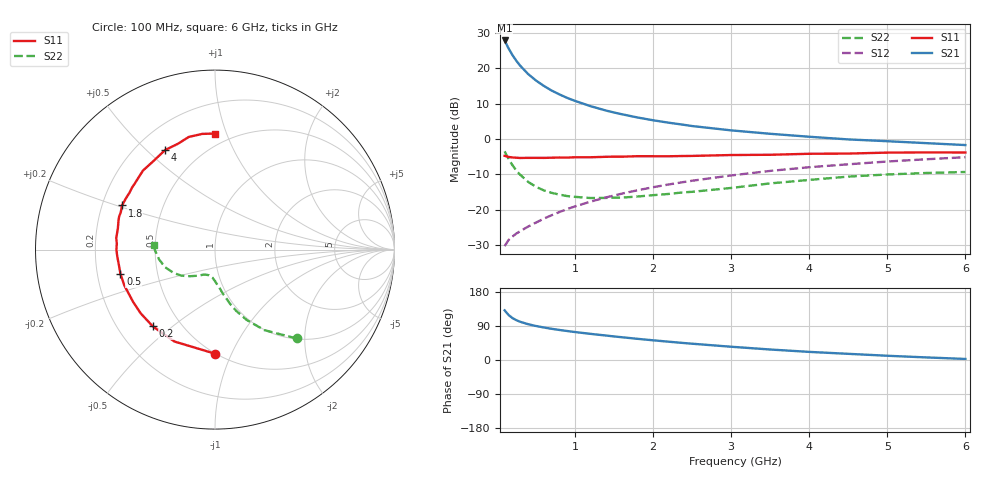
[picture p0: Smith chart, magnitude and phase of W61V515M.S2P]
! SIEMENS Small Signal Semiconductors
! BFR193W
! Si NPN RF Bipolar Junction Transistor in SOT323
! VCE = 1.5 V  IC = 15 mA
! Common Emitter S-Parameters:  September  1992
# GHz  S  MA  R  50
!  f  S11  S21  S12  S22
! GHz  MAG  ANG  MAG  ANG  MAG  ANG  MAG  ANG
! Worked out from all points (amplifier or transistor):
!   28 points, 100 MHz to 6 GHz, reference 50 ohm
!   highest |S21| = 27.9 dB at 100 MHz (marker M1)
!   |S21| within 3 dB of that: start of sweep to 170.7 MHz
!   unconditionally stable (mu >= 1): 809.9 MHz to 2.601 GHz
!   at 300 MHz: K = 0.69, MSG = 23.4 dB, |S12| = -26.0 dB
!   at 1.5 GHz: K = 1.05, MAG = 10.4 dB, |S12| = -15.9 dB
!   at 6 GHz: K = 0.92, MSG = 1.7 dB, |S12| = -5.1 dB
!   S11 on the Smith chart (normalised r, x): 100 MHz: 0.50, -0.87; 200 MHz: 0.35, -0.43; 500 MHz: 0.30, -0.12; 1.8 GHz: 0.28, +0.21; 4 GHz: 0.32, +0.57; 6 GHz: 0.41, +0.91
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0.1  0.5802 -89.9  24.77 131.1  0.0307 56.8  0.6726 -47.4
0.15  0.5598 -113.8  19.19 118.9  0.0375 52.1  0.5261 -58.5
0.2  0.5504 -129.0  15.43 110.7  0.0419 50.7  0.4291 -65.8
0.25  0.5455 -139.4  12.78 105.1  0.0463 51.1  0.359 -71.1
0.3  0.5414 -147.2  10.89 100.8  0.05 52.3  0.3128 -74.5
0.4  0.5432 -158.4  8.332 94.5  0.058 54.9  0.2495 -79.8
0.5  0.5436 -165.6  6.75 89.8  0.066 57.6  0.212 -83.6
0.6  0.5425 -171.3  5.668 85.9  0.0751 59.6  0.1891 -87.5
0.7  0.5459 -176.0  4.866 82.4  0.0838 61.2  0.1742 -90.1
0.8  0.5493 -179.9  4.291 79.3  0.0931 62.4  0.1646 -93.0
0.9  0.548 176.4  3.825 76.5  0.1026 63.3  0.1567 -95.2
1  0.5539 173.4  3.472 73.8  0.1118 63.9  0.1529 -97.5
1.2  0.5539 167.7  2.921 69.0  0.1308 64.4  0.1471 -102.9
1.5  0.5651 160.9  2.377 62.2  0.1595 64.4  0.1488 -109.5
1.8  0.5736 154.6  2.023 55.9  0.1891 63.6  0.1544 -115.1
2.2  0.5722 146.4  1.706 48.3  0.2285 61.8  0.1679 -121.2
3  0.5957 132.4  1.329 35.0  0.3064 56.5  0.2041 -133.3
3.5  0.6007 124.9  1.189 27.7  0.3554 52.5  0.2366 -142.1
4  0.6204 116.6  1.08 21.4  0.4004 48.1  0.265 -150.6
4.5  0.6245 109.4  0.99 16.3  0.4407 43.8  0.2951 -160.7
5.5  0.6485 96.3  0.877 6.8  0.519 35.1  0.3322 -178.3
6  0.6467 89.9  0.824 2.8  0.5552 30.3  0.3432 175.9
